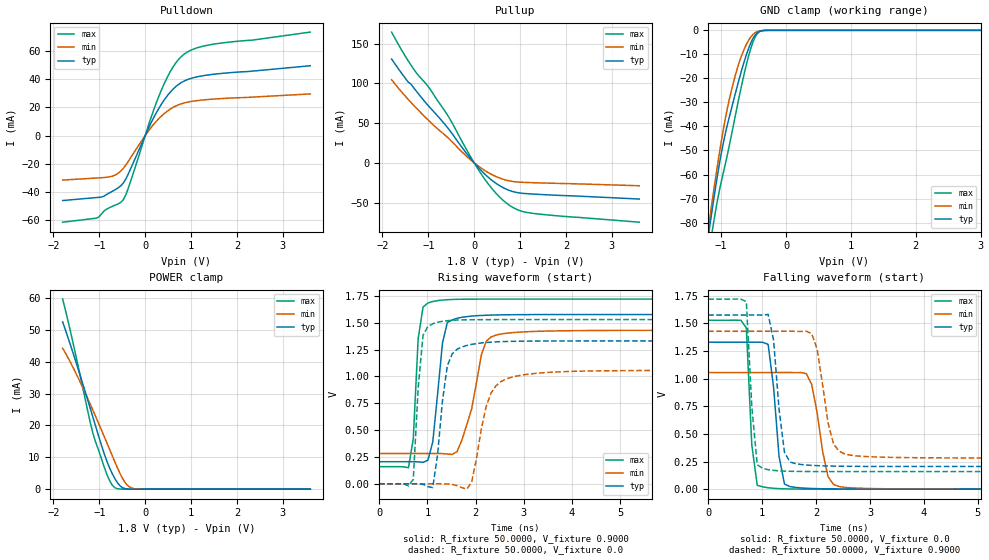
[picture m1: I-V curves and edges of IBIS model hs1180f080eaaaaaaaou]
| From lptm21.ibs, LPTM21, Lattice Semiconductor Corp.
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|   Model hs1180f080eaaaaaaaou
[Model]   hs1180f080eaaaaaaaou
Model_type   Output
Polarity   Non-Inverting
Enable   Active-Low
Vmeas =   0.9000V
Cref =   20.0000pF
Rref =   50.0000
Vref =   0.9000V
C_comp   4.2000pF   3.8000pF   7.5000pF
[Temperature Range]   25.0000   0.1050k   -40.0000
[Voltage Range]   1.8000V   1.7100V   1.8900V
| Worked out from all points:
|   slope of the pulldown table from 0 to 0.27 V, typ, clamps not added: 15.3 ohm
|   slope of the pullup table from 0 to 0.27 V, typ, clamps not added: 16.6 ohm
|   GND clamp passes 1 mA (typ) near -0.44 V on its own axis
|   POWER clamp passes 1 mA (typ) near -0.54 V on its own axis
|   rising waveform, R_fixture 50.0000, V_fixture 0.9000: 20-80 % time 180ps typ, 330ps min, 116ps max; typ from 0.205 V to 1.58 V
|   rising waveform, R_fixture 50.0000, V_fixture 0.0: 20-80 % time 193ps typ, 313ps min, 138ps max; typ from 0 V to 1.33 V
|   falling waveform, R_fixture 50.0000, V_fixture 0.0: 20-80 % time 150ps typ, 219ps min, 105ps max; typ from 1.33 V to 0 V
|   falling waveform, R_fixture 50.0000, V_fixture 0.9000: 20-80 % time 157ps typ, 228ps min, 123ps max; typ from 1.58 V to 0.205 V
[Pulldown]
|Voltage   I(typ)   I(min)   I(max)
-1.8V     -45.94mA   -31.47mA   -61.23mA
-1.02V    -43.68mA   -29.93mA   -57.79mA
-720mV    -39.44mA   -28.75mA   -50.1mA
-480mV    -33.68mA   -23.32mA   -45.45mA
-360mV    -26.52mA   -17.8mA    -36.39mA
60mV      4.338mA    2.763mA    6.157mA
360mV     22.51mA    13.97mA    32.68mA
600mV     32.57mA    19.77mA    48.13mA
840mV     38.38mA    22.95mA    57.28mA
1.08V     41.11mA    24.46mA    61.43mA
1.44V     43.12mA    25.64mA    64.3mA
3.6V      49.33mA    29.42mA    73.11mA
[Pullup]
|Voltage   I(typ)   I(min)   I(max)
-1.8V     130.8mA    104.8mA    164.8mA
-1.44V    101.9mA    80.06mA    128.7mA
-1.32V    94.74mA    72.59mA    118.2mA
-960mV    69.42mA    51.57mA    92.77mA
-600mV    45.83mA    33.12mA    61.9mA
-60mV     4.151mA    2.888mA    5.883mA
180mV     -11.32mA   -7.745mA   -16.38mA
360mV     -20.77mA   -14.04mA   -30.53mA
720mV     -33.7mA    -22.13mA   -51.5mA
960mV     -37.7mA    -24.23mA   -59.52mA
1.26V     -39.29mA   -24.99mA   -63.51mA
3.6V      -45.64mA   -28.87mA   -74.81mA
[GND_clamp]
|Voltage   I(typ)   I(min)   I(max)
-1.8V     -240.2mA   -229.4mA   -254.3mA
-1.2V     -86.16mA   -82.91mA   -94.88mA
-1.17V    -80.45mA   -77.09mA   -89.3mA
-1.11V    -69.45mA   -65.77mA   -78.87mA
-1.02V    -54.48mA   -49.86mA   -65.69mA
-930mV    -42.25mA   -35.9mA    -54.92mA
-780mV    -26.14mA   -18.58mA   -35.25mA
-690mV    -17.13mA   -10.87mA   -23.53mA
-570mV    -7.024mA   -3.834mA   -9.978mA
-450mV    -1.176mA   -584.6uA   -1.582mA
-300mV    -18.65uA   -15.9uA    -16.44uA
3.6V      0A         0A         0A
[POWER_clamp]
|Voltage   I(typ)   I(min)   I(max)
-1.8V     52.51mA    44.24mA    59.69mA
-1.68V    47.44mA    41.17mA    52.62mA
-1.5V     39.45mA    36.1mA     41.14mA
-1.26V    28.3mA     28.66mA    24.99mA
-1.14V    22.57mA    24.76mA    17.52mA
-840mV    8.928mA    14.66mA    4.779mA
-720mV    4.91mA     10.55mA    1.28mA
-660mV    3.265mA    8.507mA    435.9uA
-540mV    921.6uA    4.64mA     35.01uA
-420mV    115.2uA    1.718mA    2.184uA
-240mV    3.289uA    139.9uA    57.44nA
3.6V      -31nA      -27.04nA   -40.53nA
[Ramp]
| variable   typ   min   max
dV/dt_r  0.7825/0.1911n   0.6334/0.3102n   0.9175/0.1364n
dV/dt_f  0.8078/0.1690n   0.6265/0.2657n   0.9309/0.1315n
R_load = 50.0000
[Rising Waveform]
R_fixture=   50.0000
V_fixture=   0.9000
V_fixture_min=   0.8560
V_fixture_max=   0.9460
|time   V(typ)   V(min)   V(max)
0s        205.4mV    282.1mV    159.2mV
606.1ps   205.5mV    282.1mV    149.5mV
707.1ps   205.5mV    282.1mV    420.4mV
808.1ps   204.2mV    282.1mV    1.349V
1.01ns    219.3mV    282.1mV    1.683V
1.313ns   1.31V      281.2mV    1.711V
1.616ns   1.542V     299.4mV    1.718V
2.121ns   1.568V     1.202V     1.72V
2.424ns   1.572V     1.385V     1.72V
10ns      1.576V     1.429V     1.72V
[Rising Waveform]
R_fixture=   50.0000
V_fixture=   0.0
V_fixture_min=   0.0
V_fixture_max=   0.0
|time   V(typ)   V(min)   V(max)
0s        291.2nV    449.5nV    213.5nV
707.1ps   -66.11uV   471.6nV    41.17mV
909.1ps   -5.379mV   13.43uV    1.383V
1.111ns   -35.38mV   1.878uV    1.49V
1.414ns   1.1V       -1.561mV   1.519V
1.717ns   1.274V     -35.75mV   1.526V
1.919ns   1.299V     16.28mV    1.528V
2.323ns   1.319V     846.2mV    1.529V
2.727ns   1.326V     989.7mV    1.529V
10ns      1.33V      1.056V     1.529V
[Falling Waveform]
R_fixture=   50.0000
V_fixture=   0.0
V_fixture_min=   0.0
V_fixture_max=   0.0
|time   V(typ)   V(min)   V(max)
0s        1.33V      1.056V     1.529V
707.1ps   1.33V      1.056V     1.46V
808.1ps   1.331V     1.056V     400.6mV
909.1ps   1.331V     1.056V     34.93mV
1.111ns   1.311V     1.056V     12.68mV
1.313ns   298.2mV    1.056V     4.841mV
1.515ns   23.7mV     1.056V     1.873mV
1.919ns   6.253mV    946.7mV    286.4uV
2.424ns   1.457mV    23.95mV    46.04uV
10ns      -31.16uV   8.476uV    8.918uV
[Falling Waveform]
R_fixture=   50.0000
V_fixture=   0.9000
V_fixture_min=   0.8560
V_fixture_max=   0.9460
|time   V(typ)   V(min)   V(max)
0s        1.576V     1.429V     1.72V
707.1ps   1.576V     1.429V     1.698V
909.1ps   1.577V     1.429V     221.1mV
1.01ns    1.575V     1.429V     188.4mV
1.212ns   1.351V     1.429V     169.9mV
1.414ns   334mV      1.43V      163.3mV
1.515ns   245.8mV    1.43V      161.8mV
1.919ns   215.3mV    1.408V     159.7mV
2.525ns   207.2mV    320mV      159.3mV
10ns      205.4mV    282.1mV    159.2mV
